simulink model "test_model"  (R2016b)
settings: Solver=VariableStepAuto  StartTime=0.0  StopTime=runtime  RelTol=1e-3
InitFcn:
  | clear mex
  | delete test_model_sfun.mexw64
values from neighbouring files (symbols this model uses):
  g = 9.81    [modelParameters.m]
  height_controlled_o = (((Rm*If +      + (((omega0_o * 2 * Rm * Kv * Kq      * Kd + 1)^2) - 1)/(4* Rm*Kv^2*Kq      * Kd))/Vb)*(Pmax- Pmin) + Pmin)    [modelParameters.m]
  If = 0.511    [modelParameters.m]
  Jreq = 4.2012e-05    [modelParameters.m]
  Jxx = 0.0130    (= 0.013)    [modelParameters.m]
  Jyy = 0.0140    (= 0.014)    [modelParameters.m]
  Jzz = 0.0285    [modelParameters.m]
  Kd = 1.0317e-7    (= 1.0317e-07)    [modelParameters.m]
  Kq = 96.3422    [modelParameters.m]
  Kt = 8.6519e-6    (= 8.6519e-06)    [modelParameters.m]
  Kv = 96.3422    [modelParameters.m]
  m = 1.244    [modelParameters.m]
  omega0_o = sqrt((m*g)/(4*Kt))    [modelParameters.m]
  omega1_o = sqrt((m*g)/(4*Kt))    [modelParameters.m]
  omega2_o = sqrt((m*g)/(4*Kt))    [modelParameters.m]
  omega3_o = sqrt((m*g)/(4*Kt))    [modelParameters.m]
  pitch_o = 0    [modelParameters.m]
  pitchrate_o = 0    [modelParameters.m]
  Pmax = 2e5    (= 200000)    [modelParameters.m]
  Pmin = 1e5    (= 100000)    [modelParameters.m]
  rhx = 0.16    [modelParameters.m]
  rhy = 0.16    [modelParameters.m]
  rhz = 0.03    [modelParameters.m]
  Rm = 0.2308    [modelParameters.m]
  roll_o = 0    [modelParameters.m]
  rollrate_o = 0    [modelParameters.m]
  Tc = 0.04    [modelParameters.m]
  Tq = 0.005    [modelParameters.m]
  Vb = 11.1    [modelParameters.m]
  x_controlled_o = 0    [modelParameters.m]
  x_o = 0    [modelParameters.m]
  x_vel_o = 0    [modelParameters.m]
  y_controlled_o = 0    [modelParameters.m]
  y_o = 0    [modelParameters.m]
  y_vel_o = 0    [modelParameters.m]
  yaw_controlled_o = 0    [modelParameters.m]
  yaw_o = 0    [modelParameters.m]
  yawrate_o = 0    [modelParameters.m]
  z_o = 0    [modelParameters.m]
  z_vel_o = 0    [modelParameters.m]
undefined symbols (not defined in the file or in its folder): DiscIntNeverNeededParam
libraries: simulink x12, vrlib x2
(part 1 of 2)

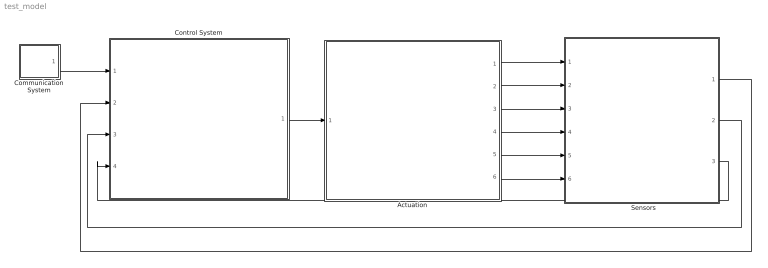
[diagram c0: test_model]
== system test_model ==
  "     Sensors   " : Subsystem
  Actuation : Subsystem
  Communication System : Subsystem
  Control System : Subsystem
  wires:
  Control System/1(P) -> Actuation/1(P)
  Communication System/1(setpoints) -> Control System/1(setpoints)
  Actuation/1(B_omega) -> "     Sensors   "/1(B_Omega)
  Actuation/2(euler_angles) -> "     Sensors   "/2(euler_angles)
  Actuation/3(B_vo) -> "     Sensors   "/3(B_vo)
  Actuation/4(E_ro) -> "     Sensors   "/4(E_ro)
  Actuation/5(B_vo_dot) -> "     Sensors   "/5(B_vo_dot)
  Actuation/6(B_g) -> "     Sensors   "/6(B_g)
  "     Sensors   "/3(current_position) -> Control System/4(current_position)
  "     Sensors   "/2(euler_rates) -> Control System/3(euler_rates)
  "     Sensors   "/1(euler_angles_filtered) -> Control System/2(euler_angles_filtered)

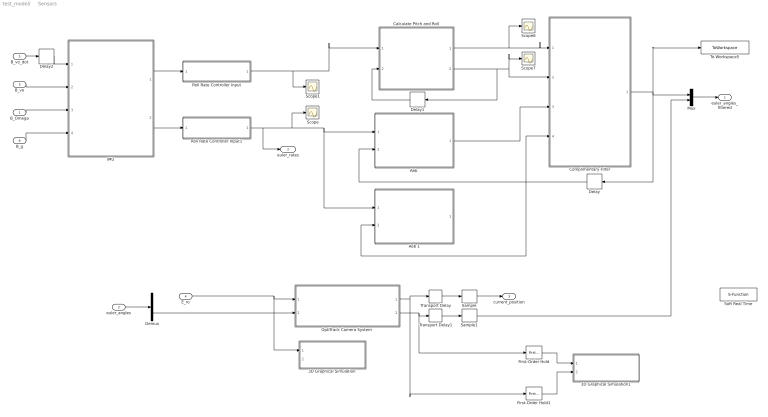
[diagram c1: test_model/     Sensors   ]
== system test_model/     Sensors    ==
  B_Omega : Inport
  euler_angles : Inport  Port=2
  B_vo : Inport  Port=3
  E_ro : Inport  Port=4
  B_vo_dot : Inport  Port=5
  B_g : Inport  Port=6
  3D Graphical Simulation : Subsystem  Commented=on
  3D Graphical Simulation1 : Subsystem  Commented=on
  "Aeb " : MATLAB Function  TreatAsAtomicUnit=on
  Aeb 1 : MATLAB Function  Commented=on  TreatAsAtomicUnit=on
  Calculate Pitch and Roll : MATLAB Function  TreatAsAtomicUnit=on
  Complimentary Filter : MATLAB Function  TreatAsAtomicUnit=on
  Delay : Delay  DelayLength=1  InitialCondition=0
  Delay1 : Delay  DelayLength=1  InitialCondition=0  SampleTime=Tq
  Delay2 : Delay  DelayLength=1  InitialCondition=0  SampleTime=Tq
  Demux : Demux  Outputs=3
  First-Order Hold : simulink/Discrete/First-Order Hold  DisableCoverage=on  Ts=5e-3
  First-Order Hold1 : simulink/Discrete/First-Order Hold  DisableCoverage=on  Ts=5e-3
  "IMU " : Subsystem
  Mux : Mux  Inputs=2
  "OptiTrack Camera System " : Subsystem
  Roll Rate Controller Input : Subsystem  Variant=on
  Roll Rate Controller Input1 : Subsystem  Variant=on
  Sample : ZeroOrderHold  SampleTime=Tc
  Sample1 : ZeroOrderHold  SampleTime=Tc
  Scope{,1,6..7} (4 alike) : Scope
  Soft Real Time : S-Function  Commented=on  FunctionName=sfun_time  Parameters=x  SFunctionDeploymentMode=off  EnableBusSupport=off
  To Workspace5 : ToWorkspace  VariableName=angle_IMU_reading  SaveFormat=Structure With Time  SampleTime=Tq
  Transport Delay : TransportDelay  DelayTime=6e-3
  Transport Delay1 : TransportDelay  DelayTime=6e-3
  euler_angles_filtered : Outport
  euler_rates : Outport  Port=2
  current_position : Outport  Port=3
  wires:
  "IMU "/1(accelerometer) -> Roll Rate Controller Input/1(raw_accel_model)
  "IMU "/2(gyroscope) -> Roll Rate Controller Input1/1(raw_gyro_model)
  B_vo/1 -> "IMU "/2(B_vo)
  B_Omega/1 -> "IMU "/3(B_Omega)
  B_g/1 -> "IMU "/4(B_g)
  Calculate Pitch and Roll/2(accel_roll) -> Scope7/1, Complimentary Filter/2(accel_roll), Delay1/1
  Calculate Pitch and Roll/1(accel_pitch) -> Scope6/1, Complimentary Filter/1(accel_pitch)
  Delay1/1 -> Calculate Pitch and Roll/2(accel_roll_prev)
  First-Order Hold/1 -> 3D Graphical Simulation1/1("Euler Angles ")
  E_ro/1 -> 3D Graphical Simulation/1(Displacement), "OptiTrack Camera System "/1(E_ro)
  First-Order Hold1/1 -> 3D Graphical Simulation1/2(Displacement)
  B_vo_dot/1 -> Delay2/1
  Delay2/1 -> "IMU "/1(B_vo_dot)
  "OptiTrack Camera System "/1(E_ro_camera) -> Transport Delay/1, First-Order Hold1/1
  "OptiTrack Camera System "/2(yaw_camera) -> First-Order Hold/1, Transport Delay1/1
  Transport Delay/1 -> Sample/1
  Transport Delay1/1 -> Sample1/1
  Sample/1 -> current_position/1
  Roll Rate Controller Input/1(raw_accel) -> Calculate Pitch and Roll/1(accel_reading), Scope1/1
  Roll Rate Controller Input1/1(raw_gyro) -> "Aeb "/1(gyro_reading), Aeb 1/1(gyro_reading), Scope/1, euler_rates/1
  Complimentary Filter/1(euler_angles_IMU) -> Mux/1, Delay/1, To Workspace5/1
  Delay/1 -> Aeb 1/2(euler_angles_filtered), Complimentary Filter/4(prev_euler_angles), "Aeb "/2(euler_angles_filtered)
  "Aeb "/1(euler_rates_IMU) -> Complimentary Filter/3(euler_rates_gyro)
  euler_angles/1 -> Demux/1
  Demux/3 -> "OptiTrack Camera System "/2(yaw)
  Sample1/1 -> Mux/2
  Mux/1 -> euler_angles_filtered/1

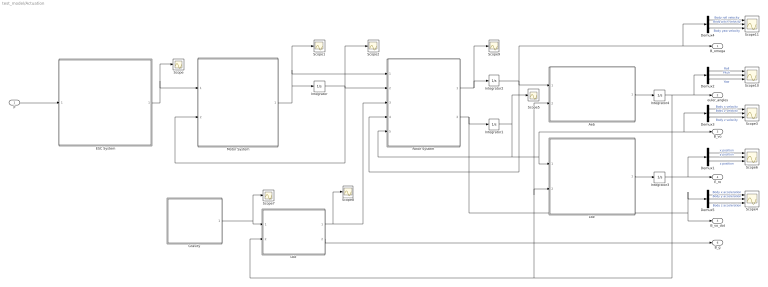
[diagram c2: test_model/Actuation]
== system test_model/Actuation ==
  P : Inport
  "Aeb " : MATLAB Function  TreatAsAtomicUnit=on
  Demux{1..5} (5 alike) : Demux  Outputs=3
  ESC System : MATLAB Function  TreatAsAtomicUnit=on
  "Gravity " : MATLAB Function  TreatAsAtomicUnit=on
  Integrator : Integrator  InitialCondition=[omega0_o, omega1_o, omega2_o, omega3_o]
  Integrator1 : Integrator  InitialCondition=[x_vel_o; y_vel_o; z_vel_o]
  Integrator2 : Integrator  InitialCondition=[rollrate_o; pitchrate_o; yawrate_o]
  Integrator3 : Integrator  InitialCondition=[x_o; y_o; z_o]
  Integrator4 : Integrator  InitialCondition=[roll_o; pitch_o; yaw_o]  ContinuousStateAttributes=['phi' 'theta' 'psi']
  "Lbe " : MATLAB Function  TreatAsAtomicUnit=on
  "Lbe " : MATLAB Function  TreatAsAtomicUnit=on
  Motor System : MATLAB Function  TreatAsAtomicUnit=on
  "Rotor System " : MATLAB Function  TreatAsAtomicUnit=on
  Scope{,1..2,5,7..9} (7 alike) : Scope
  Scope{3..4,6,10..11} (5 alike) : Scope  NumInputPorts=3
  B_omega : Outport
  euler_angles : Outport  Port=2
  B_vo : Outport  Port=3
  E_ro : Outport  Port=4
  B_vo_dot : Outport  Port=5
  B_g : Outport  Port=6
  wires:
  ESC System/1(Vb_eff) -> Scope/1, Motor System/1(Vb_eff)
  Motor System/1(w_dot) -> Integrator/1, "Rotor System "/1(w_dot), Scope1/1
  "Rotor System "/1(B_omega_dot) -> Scope9/1, Integrator2/1
  Integrator2/1 -> "Rotor System "/4(B_omega), B_omega/1, Demux4/1, "Aeb "/1(B_omega)
  "Aeb "/1(euler_rates) -> Integrator4/1
  "Lbe "/1(E_ro) -> Integrator3/1
  Integrator3/1 -> Demux1/1, E_ro/1
  "Lbe "/1(B_Fg) -> Scope8/1, "Rotor System "/3(B_Fg)
  "Lbe "/2(B_g) -> B_g/1
  Demux1/2 -> Scope6/2  "y position"
  Demux1/1 -> Scope6/1  "x position"
  Demux1/3 -> Scope6/3  "z position"
  Demux2/2 -> Scope10/2  "Pitch"
  Demux2/1 -> Scope10/1  "Roll"
  Demux2/3 -> Scope10/3  "Yaw"
  Demux4/2 -> Scope11/2  "Body pitch velocity"
  Demux4/1 -> Scope11/1  "Body roll velocity"
  Demux4/3 -> Scope11/3  "Body yaw velocity"
  Demux3/2 -> Scope3/2  "Body y velocity"
  Demux3/1 -> Scope3/1  "Body x velocity"
  Demux3/3 -> Scope3/3  "Body z velocity"
  Demux5/2 -> Scope4/2  "Body y acceleration"
  Demux5/1 -> Scope4/1  "Body x acceleration"
  Demux5/3 -> Scope4/3  "Body z acceleration"
  Integrator1/1 -> Scope5/1, "Rotor System "/5(B_vo), "Lbe "/1(B_vo), Demux3/1, B_vo/1
  "Rotor System "/2(B_vo_dot) -> Demux5/1, B_vo_dot/1, Integrator1/1
  Integrator4/1 -> euler_angles/1, Demux2/1, "Lbe "/2(euler_angles), "Aeb "/2(euler_angles), "Lbe "/2(euler_angles)
  P/1 -> ESC System/1(P)
  "Gravity "/1(E_Fg) -> Scope7/1, "Lbe "/1(E_Fg)
  Integrator/1 -> Motor System/2(w), "Rotor System "/2(w), Scope2/1

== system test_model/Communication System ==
  Step : Step  Before=[0; 0; 0; 0]  After=[0; 0; 0; 0]  SampleTime=Tq
  setpoints : Outport
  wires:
  Step/1 -> setpoints/1

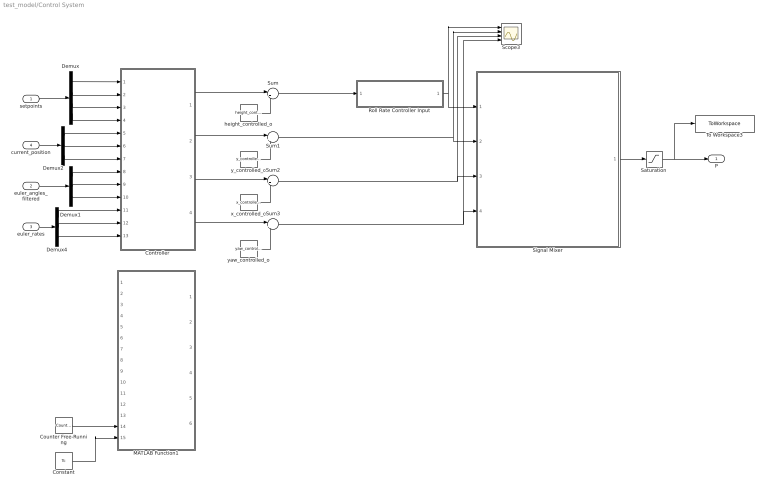
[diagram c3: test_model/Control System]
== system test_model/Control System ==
  setpoints : Inport
  euler_angles_filtered : Inport  Port=2
  euler_rates : Inport  Port=3
  current_position : Inport  Port=4
  Constant : Constant  Value=Tc  SampleTime=Tc
  Controller : Subsystem
  Counter Free-Running : simulink/Sources/Counter Free-Running  NumBits=32  tsamp=Tc
  Demux : Demux
  Demux1 : Demux  Outputs=3
  Demux2 : Demux  Outputs=3
  Demux4 : Demux  Outputs=3
  MATLAB Function1 : MATLAB Function  Commented=on  TreatAsAtomicUnit=on  SystemSampleTime=Tq
  Roll Rate Controller Input : Subsystem  Variant=on
  Saturation : Saturate  UpperLimit=Pmax*ones(4,1)  LowerLimit=Pmin*ones(4,1)
  Scope3 : Scope  NumInputPorts=4
  Signal Mixer : MATLAB Function  TreatAsAtomicUnit=on
  Sum{,1..3} (4 alike) : Sum  Inputs=|++
  To Workspace3 : ToWorkspace  VariableName=motorCommands  SaveFormat=Structure With Time  SampleTime=Tq
  height_controlled_o : Constant  Value=height_controlled_o  SampleTime=Tc
  x_controlled_o : Constant  Value=x_controlled_o
  y_controlled_o : Constant  Value=y_controlled_o
  yaw_controlled_o : Constant  Value=yaw_controlled_o
  P : Outport
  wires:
  setpoints/1 -> Demux/1
  euler_angles_filtered/1 -> Demux1/1
  current_position/1 -> Demux2/1
  euler_rates/1 -> Demux4/1
  Demux/1 -> Controller/1(x_setpoint)
  Demux/2 -> Controller/2(y_setpoint)
  Demux/3 -> Controller/3(z_setpoint)
  Demux2/1 -> Controller/5(x_position)
  Demux2/2 -> Controller/6(y_position)
  Demux2/3 -> Controller/7(z_position)
  Controller/2(y_controlled) -> Sum1/1
  Controller/4(yaw_controlled) -> Sum3/1
  y_controlled_o/1 -> Sum1/2
  x_controlled_o/1 -> Sum2/2
  yaw_controlled_o/1 -> Sum3/2
  Signal Mixer/1(P) -> Saturation/1
  Demux1/1 -> Controller/8(roll)
  Demux1/2 -> Controller/9(pitch)
  Demux4/1 -> Controller/11(roll_rate)
  Demux4/2 -> Controller/12(pitch_rate)
  Demux4/3 -> Controller/13(yaw_rate)
  Demux/4 -> Controller/4(yaw_setpoint)
  Demux1/3 -> Controller/10(yaw)
  Controller/3(x_controlled) -> Sum2/1
  Counter Free-Running/1 -> MATLAB Function1/14(vrpn_id)
  Constant/1 -> MATLAB Function1/15(Tc)
  Sum/1 -> Roll Rate Controller Input/1(z_command_model)
  height_controlled_o/1 -> Sum/2
  Saturation/1 -> To Workspace3/1, P/1
  Sum1/1 -> Scope3/2, Signal Mixer/2(y_controlled)
  Sum2/1 -> Scope3/3, Signal Mixer/3(x_controlled)
  Sum3/1 -> Scope3/4, Signal Mixer/4(yaw_controlled)
  Roll Rate Controller Input/1(z_command) -> Scope3/1, Signal Mixer/1(height_controlled)
  Controller/1(height_controlled) -> Sum/1

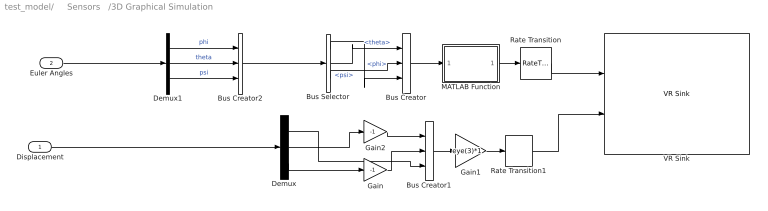
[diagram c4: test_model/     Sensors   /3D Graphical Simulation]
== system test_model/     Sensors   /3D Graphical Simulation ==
  Displacement : Inport
  Euler Angles : Inport  Port=2
  Bus Creator : BusCreator  Inputs=3
  Bus Creator1 : BusCreator  Inputs=3
  Bus Creator2 : BusCreator  Inputs=3
  Bus Selector : BusSelector  OutputSignals=phi,theta,psi
  Demux : Demux  Outputs=3
  Demux1 : Demux  Outputs=3
  Gain : Gain  Gain=-1
  Gain1 : Gain  Gain=eye(3)*1  Multiplication=Matrix(K*u)
  Gain2 : Gain  Gain=-1
  MATLAB Function : MATLAB Function  TreatAsAtomicUnit=on
  Rate Transition : RateTransition  OutPortSampleTime=0.06
  Rate Transition1 : RateTransition  OutPortSampleTime=0.06
  VR Sink : vrlib/VR Sink  InstantiateOnLoad=on  SampleTime=-1  ViewEnable=on  RemoteChange=off  RemoteView=off  FieldsWritten=Helicopter.rotation.4.1.1.double#Helicopter.translation.3.1.1.double  WorldFileName=quadrotor_world_ucart.wrl  AutoView=on  VideoDimensions=[]  AllowVariableSize=off
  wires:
  Displacement/1 -> Demux/1
  Bus Creator2/1 -> Bus Selector/1
  Demux/1 -> Bus Creator1/3
  Gain/1 -> Bus Creator1/2
  Gain2/1 -> Bus Creator1/1
  Rate Transition1/1 -> VR Sink/2
  Rate Transition/1 -> VR Sink/1
  Demux/3 -> Gain/1
  Demux/2 -> Gain2/1
  Bus Creator1/1 -> Gain1/1
  Bus Selector/1 -> Bus Creator/3  "<phi>"
  Bus Selector/3 -> Bus Creator/2  "<psi>"
  Bus Selector/2 -> Bus Creator/1  "<theta>"
  Gain1/1 -> Rate Transition1/1
  Demux1/3 -> Bus Creator2/3  "psi"
  Demux1/2 -> Bus Creator2/2  "theta"
  Demux1/1 -> Bus Creator2/1  "phi"
  Euler Angles/1 -> Demux1/1
  Bus Creator/1 -> MATLAB Function/1(u)
  MATLAB Function/1(y) -> Rate Transition/1

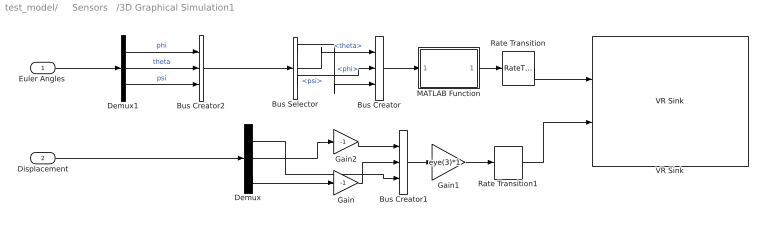
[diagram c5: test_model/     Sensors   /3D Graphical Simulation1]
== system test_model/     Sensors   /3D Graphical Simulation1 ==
  "Euler Angles " : Inport
  Displacement : Inport  Port=2
  Bus Creator : BusCreator  Inputs=3
  Bus Creator1 : BusCreator  Inputs=3
  Bus Creator2 : BusCreator  Inputs=3
  Bus Selector : BusSelector  OutputSignals=phi,theta,psi
  Demux : Demux  Outputs=3
  Demux1 : Demux  Outputs=3
  Gain : Gain  Gain=-1
  Gain1 : Gain  Gain=eye(3)*1  Multiplication=Matrix(K*u)
  Gain2 : Gain  Gain=-1
  MATLAB Function : MATLAB Function  TreatAsAtomicUnit=on
  Rate Transition : RateTransition  OutPortSampleTime=0.06
  Rate Transition1 : RateTransition  OutPortSampleTime=0.06
  VR Sink : vrlib/VR Sink  InstantiateOnLoad=on  SampleTime=-1  ViewEnable=on  RemoteChange=off  RemoteView=off  FieldsWritten=Helicopter.rotation.4.1.1.double#Helicopter.translation.3.1.1.double  WorldFileName=quadrotor_world_ucart.wrl  AutoView=on  VideoDimensions=[]  AllowVariableSize=off
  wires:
  Bus Creator2/1 -> Bus Selector/1
  Demux/1 -> Bus Creator1/3
  Gain/1 -> Bus Creator1/2
  Gain2/1 -> Bus Creator1/1
  Rate Transition1/1 -> VR Sink/2
  Rate Transition/1 -> VR Sink/1
  Demux/3 -> Gain/1
  Demux/2 -> Gain2/1
  Bus Creator1/1 -> Gain1/1
  Bus Selector/1 -> Bus Creator/3  "<phi>"
  Bus Selector/3 -> Bus Creator/2  "<psi>"
  Bus Selector/2 -> Bus Creator/1  "<theta>"
  Gain1/1 -> Rate Transition1/1
  Demux1/3 -> Bus Creator2/3  "psi"
  Demux1/2 -> Bus Creator2/2  "theta"
  Demux1/1 -> Bus Creator2/1  "phi"
  Bus Creator/1 -> MATLAB Function/1(u)
  MATLAB Function/1(y) -> Rate Transition/1
  Displacement/1 -> Demux/1
  "Euler Angles "/1 -> Demux1/1

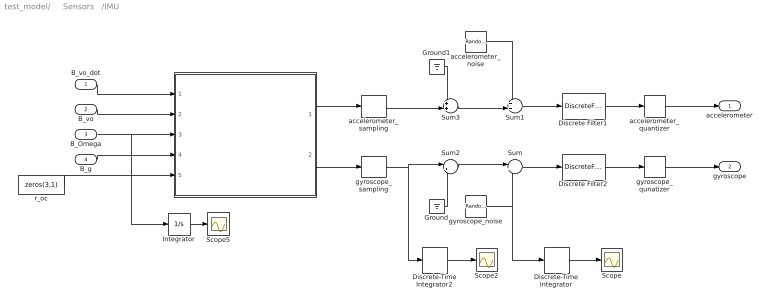
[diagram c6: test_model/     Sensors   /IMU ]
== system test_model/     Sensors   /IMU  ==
  B_vo_dot : Inport
  B_vo : Inport  Port=2
  B_Omega : Inport  Port=3
  B_g : Inport  Port=4
  " " : MATLAB Function  TreatAsAtomicUnit=on
  Discrete Filter1 : DiscreteFilter  Numerator=[0 0.1454]  Denominator=[1 -0.8546]  SampleTime=Tq
  Discrete Filter2 : DiscreteFilter  Numerator=[0 0.1454]  Denominator=[1 -0.8546]  SampleTime=Tq
  Discrete-Time Integrator : DiscreteIntegrator  InitialConditionSetting=State (most efficient)  SampleTime=-1  ICPrevOutput=DiscIntNeverNeededParam  ICPrevScaledInput=DiscIntNeverNeededParam
  Discrete-Time Integrator2 : DiscreteIntegrator  InitialConditionSetting=State (most efficient)  SampleTime=-1  ICPrevOutput=DiscIntNeverNeededParam  ICPrevScaledInput=DiscIntNeverNeededParam
  Ground : Ground
  Ground1 : Ground
  Integrator : Integrator
  Scope : Scope
  Scope2 : Scope
  Scope5 : Scope
  Sum : Sum  Inputs=|++
  Sum1 : Sum  Inputs=++|
  Sum2 : Sum  Inputs=|++
  Sum3 : Sum  Inputs=++|
  accelerometer_noise : RandomNumber  Mean=zeros(3,1)  Variance=[ 3e-7 ; 3.3e-7 ; 7.2e-7 ]  Seed=[0,1,2]  SampleTime=Tq
  accelerometer_quantizer : Quantizer  QuantizationInterval=2.4400e-04
  accelerometer_sampling : ZeroOrderHold  SampleTime=Tq
  gyroscope_noise : RandomNumber  Mean=zeros(3,1)  Variance=[ 2.2e-8 ; 1.1e-7 ; 2.4e-8 ]  Seed=[0,1,2]  SampleTime=Tq
  gyroscope_qunatizer : Quantizer  QuantizationInterval=1.1e-3
  gyroscope_sampling : ZeroOrderHold  SampleTime=Tq
  r_oc : Constant  Value=zeros(3,1)
  accelerometer : Outport
  gyroscope : Outport  Port=2
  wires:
  accelerometer_noise/1 -> Sum1/1
  Sum2/1 -> Sum/1
  Sum3/1 -> Sum1/2
  gyroscope_noise/1 -> Sum/2, Discrete-Time Integrator/1
  gyroscope_sampling/1 -> Sum2/1, Discrete-Time Integrator2/1
  accelerometer_sampling/1 -> Sum3/2
  Ground/1 -> Sum2/2
  Ground1/1 -> Sum3/1
  B_vo_dot/1 -> " "/1(B_vo_dot)
  B_vo/1 -> " "/2(B_vo)
  B_Omega/1 -> Integrator/1, " "/3(B_Omega)
  B_g/1 -> " "/4(B_g)
  r_oc/1 -> " "/5(r_oc)
  " "/2(gyroReading) -> gyroscope_sampling/1
  " "/1(accelReading) -> accelerometer_sampling/1
  Discrete-Time Integrator/1 -> Scope/1
  Discrete-Time Integrator2/1 -> Scope2/1
  Integrator/1 -> Scope5/1
  Sum1/1 -> Discrete Filter1/1
  Sum/1 -> Discrete Filter2/1
  accelerometer_quantizer/1 -> accelerometer/1
  gyroscope_qunatizer/1 -> gyroscope/1
  Discrete Filter1/1 -> accelerometer_quantizer/1
  Discrete Filter2/1 -> gyroscope_qunatizer/1

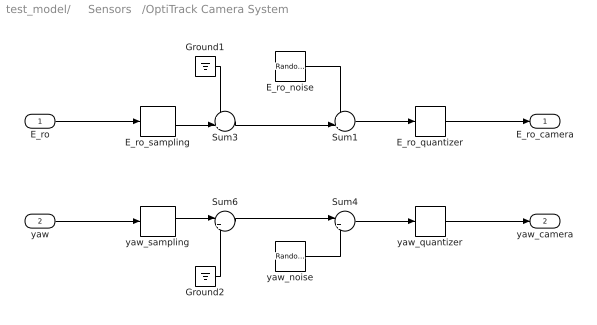
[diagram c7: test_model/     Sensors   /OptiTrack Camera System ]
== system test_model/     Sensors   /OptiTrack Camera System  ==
  E_ro : Inport
  yaw : Inport  Port=2
  E_ro_noise : RandomNumber  Mean=zeros(3,1)  Variance=[ 7.9664e-10 ; 1.1928e-10 ; 5.0636e-10 ]  Seed=[0,1,2]  SampleTime=Tc
  E_ro_quantizer : Quantizer  QuantizationInterval=2.4400e-04
  E_ro_sampling : ZeroOrderHold  SampleTime=Tc
  Ground1 : Ground
  Ground2 : Ground
  Sum1 : Sum  Inputs=++|
  Sum3 : Sum  Inputs=++|
  Sum4 : Sum  Inputs=|++
  Sum6 : Sum  Inputs=|++
  yaw_noise : RandomNumber  Variance=1.0783e-9  SampleTime=Tc
  yaw_quantizer : Quantizer  QuantizationInterval=1.1e-3
  yaw_sampling : ZeroOrderHold  SampleTime=Tc
  E_ro_camera : Outport
  yaw_camera : Outport  Port=2
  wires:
  E_ro_noise/1 -> Sum1/1
  Sum3/1 -> Sum1/2
  Sum1/1 -> E_ro_quantizer/1
  E_ro_sampling/1 -> Sum3/2
  Ground1/1 -> Sum3/1
  Sum4/1 -> yaw_quantizer/1
  Sum6/1 -> Sum4/1
  yaw_noise/1 -> Sum4/2
  yaw_sampling/1 -> Sum6/1
  Ground2/1 -> Sum6/2
  yaw/1 -> yaw_sampling/1
  E_ro/1 -> E_ro_sampling/1
  E_ro_quantizer/1 -> E_ro_camera/1
  yaw_quantizer/1 -> yaw_camera/1

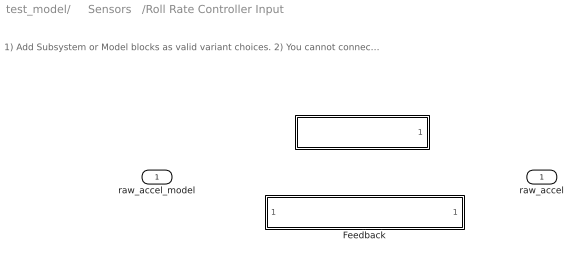
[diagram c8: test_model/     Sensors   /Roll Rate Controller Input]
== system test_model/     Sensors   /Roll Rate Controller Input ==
  note: 1) Add Subsystem or Model blocks as valid variant choices. 2) You cannot connect blocks at this level. At simulation, connectivity is automatically determined, based on the active variant and port name matching.
  raw_accel_model : Inport
  " " : Subsystem  VariantControl=logAnalysisToggle==1
  Feedback : Subsystem  VariantControl=logAnalysisToggle==0
  raw_accel : Outport

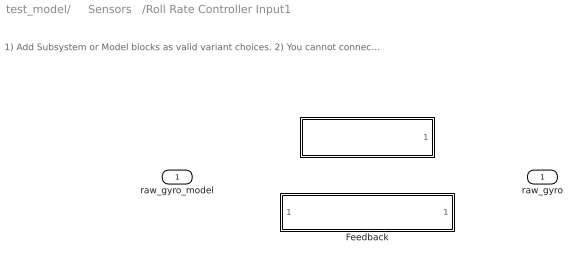
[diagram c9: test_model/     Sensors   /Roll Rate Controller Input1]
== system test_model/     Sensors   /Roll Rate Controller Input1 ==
  note: 1) Add Subsystem or Model blocks as valid variant choices. 2) You cannot connect blocks at this level. At simulation, connectivity is automatically determined, based on the active variant and port name matching.
  raw_gyro_model : Inport
  " " : Subsystem  VariantControl=logAnalysisToggle==1
  Feedback : Subsystem  VariantControl=logAnalysisToggle==0
  raw_gyro : Outport

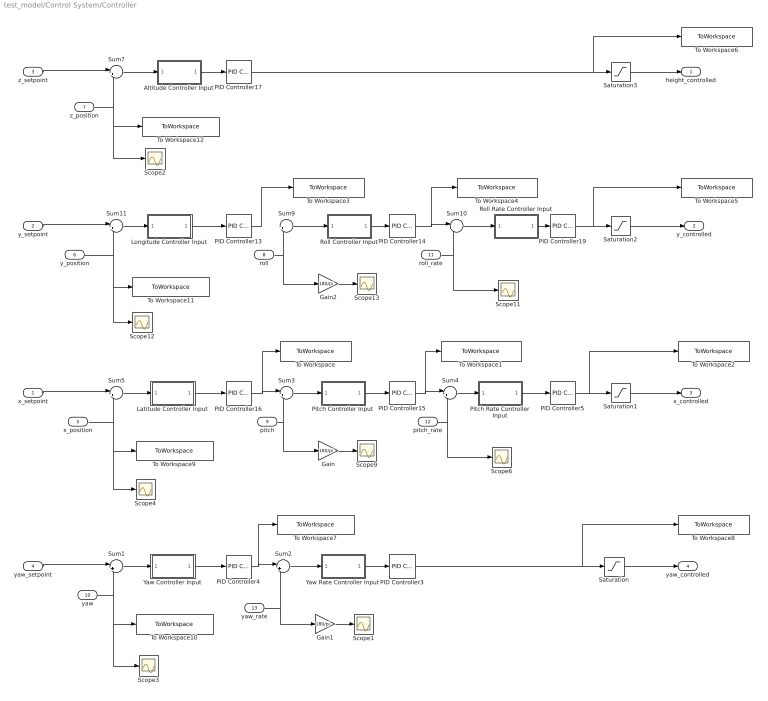
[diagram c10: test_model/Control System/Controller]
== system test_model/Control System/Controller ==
  x_setpoint : Inport
  y_setpoint : Inport  Port=2
  z_setpoint : Inport  Port=3
  yaw_setpoint : Inport  Port=4
  x_position : Inport  Port=5
  y_position : Inport  Port=6
  z_position : Inport  Port=7
  roll : Inport  Port=8
  pitch : Inport  Port=9
  yaw : Inport  Port=10
  roll_rate : Inport  Port=11
  pitch_rate : Inport  Port=12
  yaw_rate : Inport  Port=13
  Altitude Controller Input : Subsystem  Variant=on
  Gain : Gain  Gain=180/pi
  Gain1 : Gain  Gain=180/pi
  Gain2 : Gain  Gain=180/pi
  Latitude Controller Input : Subsystem  Variant=on
  Longitude Controller Input : Subsystem  Variant=on
  PID Controller13 : simulink/Continuous/PID Controller  Controller=PID  TimeDomain=Discrete-time  SampleTime=Tc  IntegratorMethod=Forward Euler  FilterMethod=Forward Euler  Form=Parallel  UseFilter=off  ControllerParametersSource=internal  P=0.015  I=0.005  D=0.03  N=33.9318377685715  InitialConditionSource=internal  InitialConditionForIntegrator=0  InitialConditionForFilter=0  ExternalReset=none  LimitOutput=off  UpperSaturationLimit=inf  LowerSaturationLimit=-inf  LinearizeAsGain=on  AntiWindupMode=none  Kb=1  TrackingMode=off  Kt=1  PParamMin=[]  PParamMax=[]  IParamMin=[]  IParamMax=[]  DParamMin=[]  DParamMax=[]  NParamMin=[]  NParamMax=[]  KbParamMin=[]  KbParamMax=[]  KtParamMin=[]  KtParamMax=[]  POutMin=[]  POutMax=[]  IOutMin=[]  IOutMax=[]  DOutMin=[]  DOutMax=[]  NOutMin=[]  NOutMax=[]  KbOutMin=[]  KbOutMax=[]  KtOutMin=[]  KtOutMax=[]  IntegratorOutMin=[]  IntegratorOutMax=[]  FilterOutMin=[]  FilterOutMax=[]  SumOutMin=[]  SumOutMax=[]  SumI1OutMin=[]  SumI1OutMax=[]  SumI2OutMin=[]  SumI2OutMax=[]  SumI3OutMin=[]  SumI3OutMax=[]  SumDOutMin=[]  SumDOutMax=[]  SaturationOutMin=[]  SaturationOutMax=[]  IntegratorContinuousStateAttributes=''  IntegratorStateMustResolveToSignalObject=off  IntegratorRTWStateStorageClass=Auto  FilterContinuousStateAttributes=''  FilterStateMustResolveToSignalObject=off  FilterRTWStateStorageClass=Auto  DifferentiatorICPrevScaledInput=0  DifferentiatorOutMin=[]  DifferentiatorOutMax=[]
  PID Controller14 : simulink/Continuous/PID Controller  Controller=PD  TimeDomain=Discrete-time  SampleTime=Tq  IntegratorMethod=Forward Euler  FilterMethod=Forward Euler  Form=Parallel  UseFilter=off  ControllerParametersSource=internal  P=15  I=35.1207902652377  D=0.2  N=40.0107970227961  InitialConditionSource=internal  InitialConditionForIntegrator=0  InitialConditionForFilter=0  ExternalReset=none  LimitOutput=off  UpperSaturationLimit=inf  LowerSaturationLimit=-inf  LinearizeAsGain=on  AntiWindupMode=none  Kb=1  TrackingMode=off  Kt=1  PParamMin=[]  PParamMax=[]  IParamMin=[]  IParamMax=[]  DParamMin=[]  DParamMax=[]  NParamMin=[]  NParamMax=[]  KbParamMin=[]  KbParamMax=[]  KtParamMin=[]  KtParamMax=[]  POutMin=[]  POutMax=[]  IOutMin=[]  IOutMax=[]  DOutMin=[]  DOutMax=[]  NOutMin=[]  NOutMax=[]  KbOutMin=[]  KbOutMax=[]  KtOutMin=[]  KtOutMax=[]  IntegratorOutMin=[]  IntegratorOutMax=[]  FilterOutMin=[]  FilterOutMax=[]  SumOutMin=[]  SumOutMax=[]  SumI1OutMin=[]  SumI1OutMax=[]  SumI2OutMin=[]  SumI2OutMax=[]  SumI3OutMin=[]  SumI3OutMax=[]  SumDOutMin=[]  SumDOutMax=[]  SaturationOutMin=[]  SaturationOutMax=[]  IntegratorContinuousStateAttributes=''  IntegratorStateMustResolveToSignalObject=off  IntegratorRTWStateStorageClass=Auto  FilterContinuousStateAttributes=''  FilterStateMustResolveToSignalObject=off  FilterRTWStateStorageClass=Auto  DifferentiatorICPrevScaledInput=0  DifferentiatorOutMin=[]  DifferentiatorOutMax=[]
  PID Controller15 : simulink/Continuous/PID Controller  Controller=PD  TimeDomain=Discrete-time  SampleTime=Tq  IntegratorMethod=Forward Euler  FilterMethod=Forward Euler  Form=Parallel  UseFilter=off  ControllerParametersSource=internal  P=15  I=35.1207902652377  D=0.2  N=40.0107970227961  InitialConditionSource=internal  InitialConditionForIntegrator=0  InitialConditionForFilter=0  ExternalReset=none  LimitOutput=off  UpperSaturationLimit=inf  LowerSaturationLimit=-inf  LinearizeAsGain=on  AntiWindupMode=none  Kb=1  TrackingMode=off  Kt=1  PParamMin=[]  PParamMax=[]  IParamMin=[]  IParamMax=[]  DParamMin=[]  DParamMax=[]  NParamMin=[]  NParamMax=[]  KbParamMin=[]  KbParamMax=[]  KtParamMin=[]  KtParamMax=[]  POutMin=[]  POutMax=[]  IOutMin=[]  IOutMax=[]  DOutMin=[]  DOutMax=[]  NOutMin=[]  NOutMax=[]  KbOutMin=[]  KbOutMax=[]  KtOutMin=[]  KtOutMax=[]  IntegratorOutMin=[]  IntegratorOutMax=[]  FilterOutMin=[]  FilterOutMax=[]  SumOutMin=[]  SumOutMax=[]  SumI1OutMin=[]  SumI1OutMax=[]  SumI2OutMin=[]  SumI2OutMax=[]  SumI3OutMin=[]  SumI3OutMax=[]  SumDOutMin=[]  SumDOutMax=[]  SaturationOutMin=[]  SaturationOutMax=[]  IntegratorContinuousStateAttributes=''  IntegratorStateMustResolveToSignalObject=off  IntegratorRTWStateStorageClass=Auto  FilterContinuousStateAttributes=''  FilterStateMustResolveToSignalObject=off  FilterRTWStateStorageClass=Auto  DifferentiatorICPrevScaledInput=0  DifferentiatorOutMin=[]  DifferentiatorOutMax=[]
  PID Controller16 : simulink/Continuous/PID Controller  Controller=PID  TimeDomain=Discrete-time  SampleTime=Tc  IntegratorMethod=Forward Euler  FilterMethod=Forward Euler  Form=Parallel  UseFilter=off  ControllerParametersSource=internal  P=-0.015  I=-0.005  D=-0.03  N=33.9318377685715  InitialConditionSource=internal  InitialConditionForIntegrator=0  InitialConditionForFilter=0  ExternalReset=none  LimitOutput=off  UpperSaturationLimit=inf  LowerSaturationLimit=-inf  LinearizeAsGain=on  AntiWindupMode=none  Kb=1  TrackingMode=off  Kt=1  PParamMin=[]  PParamMax=[]  IParamMin=[]  IParamMax=[]  DParamMin=[]  DParamMax=[]  NParamMin=[]  NParamMax=[]  KbParamMin=[]  KbParamMax=[]  KtParamMin=[]  KtParamMax=[]  POutMin=[]  POutMax=[]  IOutMin=[]  IOutMax=[]  DOutMin=[]  DOutMax=[]  NOutMin=[]  NOutMax=[]  KbOutMin=[]  KbOutMax=[]  KtOutMin=[]  KtOutMax=[]  IntegratorOutMin=[]  IntegratorOutMax=[]  FilterOutMin=[]  FilterOutMax=[]  SumOutMin=[]  SumOutMax=[]  SumI1OutMin=[]  SumI1OutMax=[]  SumI2OutMin=[]  SumI2OutMax=[]  SumI3OutMin=[]  SumI3OutMax=[]  SumDOutMin=[]  SumDOutMax=[]  SaturationOutMin=[]  SaturationOutMax=[]  IntegratorContinuousStateAttributes=''  IntegratorStateMustResolveToSignalObject=off  IntegratorRTWStateStorageClass=Auto  FilterContinuousStateAttributes=''  FilterStateMustResolveToSignalObject=off  FilterRTWStateStorageClass=Auto  DifferentiatorICPrevScaledInput=0  DifferentiatorOutMin=[]  DifferentiatorOutMax=[]
  PID Controller17 : simulink/Continuous/PID Controller  Controller=PID  TimeDomain=Discrete-time  SampleTime=Tc  IntegratorMethod=Forward Euler  FilterMethod=Forward Euler  Form=Parallel  UseFilter=off  ControllerParametersSource=internal  P=9804  I=817  D=7353  N=5.79502261645411  InitialConditionSource=internal  InitialConditionForIntegrator=0  InitialConditionForFilter=0  ExternalReset=none  LimitOutput=off  UpperSaturationLimit=inf  LowerSaturationLimit=-inf  LinearizeAsGain=on  AntiWindupMode=none  Kb=1  TrackingMode=off  Kt=1  PParamMin=[]  PParamMax=[]  IParamMin=[]  IParamMax=[]  DParamMin=[]  DParamMax=[]  NParamMin=[]  NParamMax=[]  KbParamMin=[]  KbParamMax=[]  KtParamMin=[]  KtParamMax=[]  POutMin=[]  POutMax=[]  IOutMin=[]  IOutMax=[]  DOutMin=[]  DOutMax=[]  NOutMin=[]  NOutMax=[]  KbOutMin=[]  KbOutMax=[]  KtOutMin=[]  KtOutMax=[]  IntegratorOutMin=[]  IntegratorOutMax=[]  FilterOutMin=[]  FilterOutMax=[]  SumOutMin=[]  SumOutMax=[]  SumI1OutMin=[]  SumI1OutMax=[]  SumI2OutMin=[]  SumI2OutMax=[]  SumI3OutMin=[]  SumI3OutMax=[]  SumDOutMin=[]  SumDOutMax=[]  SaturationOutMin=[]  SaturationOutMax=[]  IntegratorContinuousStateAttributes=''  IntegratorStateMustResolveToSignalObject=off  IntegratorRTWStateStorageClass=Auto  FilterContinuousStateAttributes=''  FilterStateMustResolveToSignalObject=off  FilterRTWStateStorageClass=Auto  DifferentiatorICPrevScaledInput=0  DifferentiatorOutMin=[]  DifferentiatorOutMax=[]
  PID Controller19 : simulink/Continuous/PID Controller  Controller=PD  TimeDomain=Discrete-time  SampleTime=Tq  IntegratorMethod=Forward Euler  FilterMethod=Forward Euler  Form=Parallel  UseFilter=off  ControllerParametersSource=internal  P=4600  I=1575.82088970639  D=550  N=244.660686071579  InitialConditionSource=internal  InitialConditionForIntegrator=0  InitialConditionForFilter=0  ExternalReset=none  LimitOutput=off  UpperSaturationLimit=inf  LowerSaturationLimit=-inf  LinearizeAsGain=on  AntiWindupMode=none  Kb=1  TrackingMode=off  Kt=1  PParamMin=[]  PParamMax=[]  IParamMin=[]  IParamMax=[]  DParamMin=[]  DParamMax=[]  NParamMin=[]  NParamMax=[]  KbParamMin=[]  KbParamMax=[]  KtParamMin=[]  KtParamMax=[]  POutMin=[]  POutMax=[]  IOutMin=[]  IOutMax=[]  DOutMin=[]  DOutMax=[]  NOutMin=[]  NOutMax=[]  KbOutMin=[]  KbOutMax=[]  KtOutMin=[]  KtOutMax=[]  IntegratorOutMin=[]  IntegratorOutMax=[]  FilterOutMin=[]  FilterOutMax=[]  SumOutMin=[]  SumOutMax=[]  SumI1OutMin=[]  SumI1OutMax=[]  SumI2OutMin=[]  SumI2OutMax=[]  SumI3OutMin=[]  SumI3OutMax=[]  SumDOutMin=[]  SumDOutMax=[]  SaturationOutMin=[]  SaturationOutMax=[]  IntegratorContinuousStateAttributes=''  IntegratorStateMustResolveToSignalObject=off  IntegratorRTWStateStorageClass=Auto  FilterContinuousStateAttributes=''  FilterStateMustResolveToSignalObject=off  FilterRTWStateStorageClass=Auto  DifferentiatorICPrevScaledInput=0  DifferentiatorOutMin=[]  DifferentiatorOutMax=[]
  PID Controller3 : simulink/Continuous/PID Controller  Controller=P  TimeDomain=Discrete-time  SampleTime=Tq  IntegratorMethod=Forward Euler  FilterMethod=Forward Euler  Form=Parallel  UseFilter=on  ControllerParametersSource=internal  P=435480  I=-77.7  D=2.32  N=1/0.0818  InitialConditionSource=internal  InitialConditionForIntegrator=0  InitialConditionForFilter=0  ExternalReset=none  ZeroCross=off  LimitOutput=off  UpperSaturationLimit=inf  LowerSaturationLimit=-inf  LinearizeAsGain=on  AntiWindupMode=none  Kb=1  TrackingMode=off  Kt=1  PParamMin=[]  PParamMax=[]  IParamMin=[]  IParamMax=[]  DParamMin=[]  DParamMax=[]  NParamMin=[]  NParamMax=[]  KbParamMin=[]  KbParamMax=[]  KtParamMin=[]  KtParamMax=[]  POutMin=[]  POutMax=[]  IOutMin=[]  IOutMax=[]  DOutMin=[]  DOutMax=[]  NOutMin=[]  NOutMax=[]  KbOutMin=[]  KbOutMax=[]  KtOutMin=[]  KtOutMax=[]  IntegratorOutMin=[]  IntegratorOutMax=[]  FilterOutMin=[]  FilterOutMax=[]  SumOutMin=[]  SumOutMax=[]  SumI1OutMin=[]  SumI1OutMax=[]  SumI2OutMin=[]  SumI2OutMax=[]  SumI3OutMin=[]  SumI3OutMax=[]  SumDOutMin=[]  SumDOutMax=[]  SaturationOutMin=[]  SaturationOutMax=[]  IntegratorContinuousStateAttributes=''  IntegratorStateMustResolveToSignalObject=off  IntegratorRTWStateStorageClass=Auto  FilterContinuousStateAttributes=''  FilterStateMustResolveToSignalObject=off  FilterRTWStateStorageClass=Auto  DifferentiatorICPrevScaledInput=0  DifferentiatorOutMin=[]  DifferentiatorOutMax=[]
  PID Controller4 : simulink/Continuous/PID Controller  Controller=PD  TimeDomain=Discrete-time  SampleTime=Tc  IntegratorMethod=Forward Euler  FilterMethod=Forward Euler  Form=Parallel  UseFilter=off  ControllerParametersSource=internal  P=2.6  I=2.36803176515497  D=0  N=3.83298618768959  InitialConditionSource=internal  InitialConditionForIntegrator=0  InitialConditionForFilter=0  ExternalReset=none  LimitOutput=off  UpperSaturationLimit=inf  LowerSaturationLimit=-inf  LinearizeAsGain=on  AntiWindupMode=none  Kb=1  TrackingMode=off  Kt=1  PParamMin=[]  PParamMax=[]  IParamMin=[]  IParamMax=[]  DParamMin=[]  DParamMax=[]  NParamMin=[]  NParamMax=[]  KbParamMin=[]  KbParamMax=[]  KtParamMin=[]  KtParamMax=[]  POutMin=[]  POutMax=[]  IOutMin=[]  IOutMax=[]  DOutMin=[]  DOutMax=[]  NOutMin=[]  NOutMax=[]  KbOutMin=[]  KbOutMax=[]  KtOutMin=[]  KtOutMax=[]  IntegratorOutMin=[]  IntegratorOutMax=[]  FilterOutMin=[]  FilterOutMax=[]  SumOutMin=[]  SumOutMax=[]  SumI1OutMin=[]  SumI1OutMax=[]  SumI2OutMin=[]  SumI2OutMax=[]  SumI3OutMin=[]  SumI3OutMax=[]  SumDOutMin=[]  SumDOutMax=[]  SaturationOutMin=[]  SaturationOutMax=[]  IntegratorContinuousStateAttributes=''  IntegratorStateMustResolveToSignalObject=off  IntegratorRTWStateStorageClass=Auto  FilterContinuousStateAttributes=''  FilterStateMustResolveToSignalObject=off  FilterRTWStateStorageClass=Auto  DifferentiatorICPrevScaledInput=0  DifferentiatorOutMin=[]  DifferentiatorOutMax=[]
  PID Controller5 : simulink/Continuous/PID Controller  Controller=PD  TimeDomain=Discrete-time  SampleTime=Tq  IntegratorMethod=Forward Euler  FilterMethod=Forward Euler  Form=Parallel  UseFilter=off  ControllerParametersSource=internal  P=4600  I=1575.82088970639  D=550  N=244.660686071579  InitialConditionSource=internal  InitialConditionForIntegrator=0  InitialConditionForFilter=0  ExternalReset=none  LimitOutput=off  UpperSaturationLimit=inf  LowerSaturationLimit=-inf  LinearizeAsGain=on  AntiWindupMode=none  Kb=1  TrackingMode=off  Kt=1  PParamMin=[]  PParamMax=[]  IParamMin=[]  IParamMax=[]  DParamMin=[]  DParamMax=[]  NParamMin=[]  NParamMax=[]  KbParamMin=[]  KbParamMax=[]  KtParamMin=[]  KtParamMax=[]  POutMin=[]  POutMax=[]  IOutMin=[]  IOutMax=[]  DOutMin=[]  DOutMax=[]  NOutMin=[]  NOutMax=[]  KbOutMin=[]  KbOutMax=[]  KtOutMin=[]  KtOutMax=[]  IntegratorOutMin=[]  IntegratorOutMax=[]  FilterOutMin=[]  FilterOutMax=[]  SumOutMin=[]  SumOutMax=[]  SumI1OutMin=[]  SumI1OutMax=[]  SumI2OutMin=[]  SumI2OutMax=[]  SumI3OutMin=[]  SumI3OutMax=[]  SumDOutMin=[]  SumDOutMax=[]  SaturationOutMin=[]  SaturationOutMax=[]  IntegratorContinuousStateAttributes=''  IntegratorStateMustResolveToSignalObject=off  IntegratorRTWStateStorageClass=Auto  FilterContinuousStateAttributes=''  FilterStateMustResolveToSignalObject=off  FilterRTWStateStorageClass=Auto  DifferentiatorICPrevScaledInput=0  DifferentiatorOutMin=[]  DifferentiatorOutMax=[]
  Pitch Controller Input : Subsystem  Variant=on
  Pitch Rate Controller Input : Subsystem  Variant=on
  Roll Controller Input : Subsystem  Variant=on
  Roll Rate Controller Input : Subsystem  Variant=on
  Saturation{,1..3} (4 alike) : Saturate  UpperLimit=30000  LowerLimit=-30000
  Scope{1..4,6,9,11..13} (9 alike) : Scope
  Sum{1..5,7,9..11} (9 alike) : Sum  Inputs=|+-
  To Workspace : ToWorkspace  VariableName=pitch_setpoint_model  SaveFormat=Structure With Time  SampleTime=-1
  To Workspace1 : ToWorkspace  VariableName=pitchrate_setpoint_model  SaveFormat=Structure With Time  SampleTime=Tq
  To Workspace10 : ToWorkspace  VariableName=yaw_value_model  SaveFormat=Structure With Time  SampleTime=Tc
  To Workspace11 : ToWorkspace  VariableName=y_position_model  SaveFormat=Structure With Time  SampleTime=Tc
  To Workspace12 : ToWorkspace  VariableName=z_position_model  SaveFormat=Structure With Time  SampleTime=Tc
  To Workspace2 : ToWorkspace  VariableName=x_command_model  SaveFormat=Structure With Time  SampleTime=Tq
  To Workspace3 : ToWorkspace  VariableName=roll_setpoint_model  SaveFormat=Structure With Time  SampleTime=Tc
  To Workspace4 : ToWorkspace  VariableName=rollrate_setpoint_model  SaveFormat=Structure With Time  SampleTime=Tq
  To Workspace5 : ToWorkspace  VariableName=y_command_model  SaveFormat=Structure With Time  SampleTime=Tq
  To Workspace6 : ToWorkspace  VariableName=z_command_model  SaveFormat=Structure With Time  SampleTime=Tc
  To Workspace7 : ToWorkspace  VariableName=yawrate_setpoint_model  SaveFormat=Structure With Time  SampleTime=Tc
  To Workspace8 : ToWorkspace  VariableName=yaw_command_model  SaveFormat=Structure With Time  SampleTime=Tq
  To Workspace9 : ToWorkspace  VariableName=x_position_model  SaveFormat=Structure With Time  SampleTime=Tc
  Yaw Controller Input : Subsystem  Variant=on
  Yaw Rate Controller Input : Subsystem  Variant=on
  height_controlled : Outport
  y_controlled : Outport  Port=2
  x_controlled : Outport  Port=3
  yaw_controlled : Outport  Port=4
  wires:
  pitch_rate/1 -> Scope6/1, Sum4/2
  z_setpoint/1 -> Sum7/1
  x_position/1 -> Scope4/1, To Workspace9/1, Sum5/2
  PID Controller15/1 -> Sum4/1, To Workspace1/1
  PID Controller16/1 -> Sum3/1, To Workspace/1
  pitch/1 -> Gain/1, Sum3/2
  Gain/1 -> Scope9/1
  PID Controller3/1 -> To Workspace8/1, Saturation/1
  PID Controller5/1 -> To Workspace2/1, Saturation1/1
  Latitude Controller Input/1(x_error) -> PID Controller16/1
  x_setpoint/1 -> Sum5/1
  roll_rate/1 -> Scope11/1, Sum10/2
  y_position/1 -> Scope12/1, To Workspace11/1, Sum11/2
  PID Controller14/1 -> Sum10/1, To Workspace4/1
  PID Controller13/1 -> To Workspace3/1
  roll/1 -> Gain2/1, Sum9/2
  Gain2/1 -> Scope13/1
  PID Controller19/1 -> To Workspace5/1, Saturation2/1
  y_setpoint/1 -> Sum11/1
  PID Controller17/1 -> To Workspace6/1, Saturation3/1
  yaw/1 -> Scope3/1, To Workspace10/1, Sum1/2
  yaw_setpoint/1 -> Sum1/1
  yaw_rate/1 -> Gain1/1, Sum2/2
  Gain1/1 -> Scope1/1
  PID Controller4/1 -> To Workspace7/1, Sum2/1
  z_position/1 -> To Workspace12/1, Scope2/1, Sum7/2
  Sum1/1 -> Yaw Controller Input/1(yaw_error_model)
  Yaw Controller Input/1(yaw_error) -> PID Controller4/1
  Sum2/1 -> Yaw Rate Controller Input/1(yawrate_error_model)
  Yaw Rate Controller Input/1(yawrate_error) -> PID Controller3/1
  Sum5/1 -> Latitude Controller Input/1(x_error_model)
  Sum3/1 -> Pitch Controller Input/1(pitch_error_model)
  Pitch Controller Input/1(pitch_error) -> PID Controller15/1
  Sum4/1 -> Pitch Rate Controller Input/1(pitchrate_error_model)
  Pitch Rate Controller Input/1(pitchrate_error) -> PID Controller5/1
  Sum11/1 -> Longitude Controller Input/1(y_error_model)
  Longitude Controller Input/1(y_error) -> PID Controller13/1
  Sum9/1 -> Roll Controller Input/1(roll_error_model)
  Roll Controller Input/1(roll_error) -> PID Controller14/1
  Sum10/1 -> Roll Rate Controller Input/1(rollrate_error_model)
  Roll Rate Controller Input/1(rollrate_error) -> PID Controller19/1
  Altitude Controller Input/1(z_error) -> PID Controller17/1
  Sum7/1 -> Altitude Controller Input/1(z_error_model)
  Saturation2/1 -> y_controlled/1
  Saturation3/1 -> height_controlled/1
  Saturation1/1 -> x_controlled/1
  Saturation/1 -> yaw_controlled/1

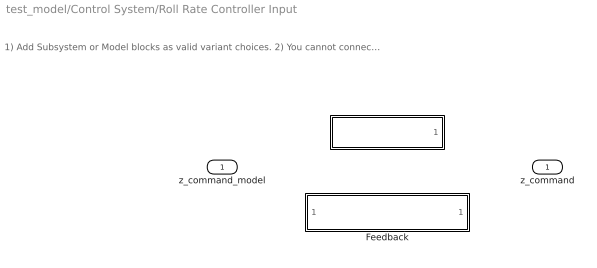
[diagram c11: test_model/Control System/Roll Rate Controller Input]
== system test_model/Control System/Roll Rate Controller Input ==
  note: 1) Add Subsystem or Model blocks as valid variant choices. 2) You cannot connect blocks at this level. At simulation, connectivity is automatically determined, based on the active variant and port name matching.
  z_command_model : Inport
  " " : Subsystem  VariantControl=logAnalysisToggle==1
  Feedback : Subsystem  VariantControl=logAnalysisToggle==0
  z_command : Outport

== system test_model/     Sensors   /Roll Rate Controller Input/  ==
  From Workspace5 : FromWorkspace  VariableName=raw_accel_data  SampleTime=Tq
  raw_accel : Outport
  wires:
  From Workspace5/1 -> raw_accel/1

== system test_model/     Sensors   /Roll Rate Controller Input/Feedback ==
  raw_accel_model : Inport
  raw_accel : Outport
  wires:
  raw_accel_model/1 -> raw_accel/1

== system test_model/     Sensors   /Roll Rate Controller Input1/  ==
  From Workspace5 : FromWorkspace  VariableName=raw_accel_data  SampleTime=Tq
  raw_gyro : Outport
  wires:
  From Workspace5/1 -> raw_gyro/1

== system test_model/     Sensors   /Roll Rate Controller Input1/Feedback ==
  raw_gyro_model : Inport
  raw_gyro : Outport
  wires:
  raw_gyro_model/1 -> raw_gyro/1

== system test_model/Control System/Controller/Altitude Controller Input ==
  note: 1) Add Subsystem or Model blocks as valid variant choices. 2) You cannot connect blocks at this level. At simulation, connectivity is automatically determined, based on the active variant and port name matching.
  z_error_model : Inport
  Feedback : Subsystem  VariantControl=logAnalysisToggle==0
  z error : Subsystem  VariantControl=logAnalysisToggle==1
  z_error : Outport

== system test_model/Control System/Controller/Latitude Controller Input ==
  note: 1) Add Subsystem or Model blocks as valid variant choices. 2) You cannot connect blocks at this level. At simulation, connectivity is automatically determined, based on the active variant and port name matching.
  x_error_model : Inport
  Feedback : Subsystem  VariantControl=logAnalysisToggle==0
  x error : Subsystem  VariantControl=logAnalysisToggle==1
  x_error : Outport

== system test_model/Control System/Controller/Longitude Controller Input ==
  note: 1) Add Subsystem or Model blocks as valid variant choices. 2) You cannot connect blocks at this level. At simulation, connectivity is automatically determined, based on the active variant and port name matching.
  y_error_model : Inport
  Feedback : Subsystem  VariantControl=logAnalysisToggle==0
  y error : Subsystem  VariantControl=logAnalysisToggle==1
  y_error : Outport

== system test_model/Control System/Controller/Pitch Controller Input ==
  note: 1) Add Subsystem or Model blocks as valid variant choices. 2) You cannot connect blocks at this level. At simulation, connectivity is automatically determined, based on the active variant and port name matching.
  pitch_error_model : Inport
  Feedback : Subsystem  VariantControl=logAnalysisToggle==0
  pitch error : Subsystem  VariantControl=logAnalysisToggle==1
  pitch_error : Outport

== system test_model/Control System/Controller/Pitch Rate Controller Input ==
  note: 1) Add Subsystem or Model blocks as valid variant choices. 2) You cannot connect blocks at this level. At simulation, connectivity is automatically determined, based on the active variant and port name matching.
  pitchrate_error_model : Inport
  Feedback : Subsystem  VariantControl=logAnalysisToggle==0
  pitchrate error : Subsystem  VariantControl=logAnalysisToggle==1
  pitchrate_error : Outport

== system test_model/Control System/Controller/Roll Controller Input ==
  note: 1) Add Subsystem or Model blocks as valid variant choices. 2) You cannot connect blocks at this level. At simulation, connectivity is automatically determined, based on the active variant and port name matching.
  roll_error_model : Inport
  Feedback : Subsystem  VariantControl=logAnalysisToggle==0
  roll error : Subsystem  VariantControl=logAnalysisToggle==1
  roll_error : Outport

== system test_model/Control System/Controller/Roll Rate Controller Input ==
  note: 1) Add Subsystem or Model blocks as valid variant choices. 2) You cannot connect blocks at this level. At simulation, connectivity is automatically determined, based on the active variant and port name matching.
  rollrate_error_model : Inport
  Feedback : Subsystem  VariantControl=logAnalysisToggle==0
  rollrate error : Subsystem  VariantControl=logAnalysisToggle==1
  rollrate_error : Outport

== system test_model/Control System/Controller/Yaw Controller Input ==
  note: 1) Add Subsystem or Model blocks as valid variant choices. 2) You cannot connect blocks at this level. At simulation, connectivity is automatically determined, based on the active variant and port name matching.
  yaw_error_model : Inport
  Feedback : Subsystem  VariantControl=logAnalysisToggle==0
  yaw error : Subsystem  VariantControl=logAnalysisToggle==1
  yaw_error : Outport

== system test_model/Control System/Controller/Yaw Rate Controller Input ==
  note: 1) Add Subsystem or Model blocks as valid variant choices. 2) You cannot connect blocks at this level. At simulation, connectivity is automatically determined, based on the active variant and port name matching.
  yawrate_error_model : Inport
  Feedback : Subsystem  VariantControl=logAnalysisToggle==0
  yawrate error : Subsystem  VariantControl=logAnalysisToggle==1
  yawrate_error : Outport

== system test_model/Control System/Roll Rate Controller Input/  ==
  From Workspace5 : FromWorkspace  VariableName=throttle_command  SampleTime=Tq
  z_command : Outport
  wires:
  From Workspace5/1 -> z_command/1

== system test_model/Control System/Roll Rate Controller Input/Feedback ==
  z_command_model : Inport
  z_command : Outport
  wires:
  z_command_model/1 -> z_command/1

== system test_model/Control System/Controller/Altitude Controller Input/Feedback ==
  z_error_model : Inport
  z_error : Outport
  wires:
  z_error_model/1 -> z_error/1

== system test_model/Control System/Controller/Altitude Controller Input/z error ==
  From Workspace6 : FromWorkspace  VariableName=z_error  SampleTime=Tc
  z_error : Outport
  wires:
  From Workspace6/1 -> z_error/1

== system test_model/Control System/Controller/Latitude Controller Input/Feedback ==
  x_error_model : Inport
  x_error : Outport
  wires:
  x_error_model/1 -> x_error/1

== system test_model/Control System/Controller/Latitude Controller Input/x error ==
  From Workspace : FromWorkspace  VariableName=x_error  SampleTime=Tc
  x_error : Outport
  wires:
  From Workspace/1 -> x_error/1

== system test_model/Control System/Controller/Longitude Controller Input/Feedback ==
  y_error_model : Inport
  y_error : Outport
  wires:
  y_error_model/1 -> y_error/1

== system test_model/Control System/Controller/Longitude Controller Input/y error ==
  From Workspace3 : FromWorkspace  VariableName=y_error  SampleTime=Tc
  y_error : Outport
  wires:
  From Workspace3/1 -> y_error/1

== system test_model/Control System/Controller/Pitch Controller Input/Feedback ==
  pitch_error_model : Inport
  pitch_error : Outport
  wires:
  pitch_error_model/1 -> pitch_error/1

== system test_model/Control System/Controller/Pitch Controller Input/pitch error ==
  From Workspace : FromWorkspace  VariableName=pitch_error  SampleTime=Tq
  pitch_error : Outport
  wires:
  From Workspace/1 -> pitch_error/1

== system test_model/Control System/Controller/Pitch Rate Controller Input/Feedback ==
  pitchrate_error_model : Inport
  pitchrate_error : Outport
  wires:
  pitchrate_error_model/1 -> pitchrate_error/1

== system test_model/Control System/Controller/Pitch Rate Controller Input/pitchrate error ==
  From Workspace2 : FromWorkspace  VariableName=pitchrate_error  SampleTime=Tq
  pitchrate_error : Outport
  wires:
  From Workspace2/1 -> pitchrate_error/1

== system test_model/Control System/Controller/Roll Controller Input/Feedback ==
  roll_error_model : Inport
  roll_error : Outport
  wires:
  roll_error_model/1 -> roll_error/1

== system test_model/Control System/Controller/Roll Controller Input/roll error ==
  From Workspace4 : FromWorkspace  VariableName=roll_error  SampleTime=Tq
  roll_error : Outport
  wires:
  From Workspace4/1 -> roll_error/1

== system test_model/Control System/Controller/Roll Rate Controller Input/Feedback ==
  rollrate_error_model : Inport
  rollrate_error : Outport
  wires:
  rollrate_error_model/1 -> rollrate_error/1

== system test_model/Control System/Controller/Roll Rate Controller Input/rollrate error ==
  From Workspace5 : FromWorkspace  VariableName=rollrate_error  SampleTime=Tq
  rollrate_error : Outport
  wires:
  From Workspace5/1 -> rollrate_error/1

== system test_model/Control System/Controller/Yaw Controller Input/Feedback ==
  yaw_error_model : Inport
  yaw_error : Outport
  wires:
  yaw_error_model/1 -> yaw_error/1

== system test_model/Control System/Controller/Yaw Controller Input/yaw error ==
  From Workspace7 : FromWorkspace  VariableName=yaw_error  SampleTime=Tc
  yaw_error : Outport
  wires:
  From Workspace7/1 -> yaw_error/1

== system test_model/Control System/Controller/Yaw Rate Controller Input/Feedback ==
  yawrate_error_model : Inport
  yawrate_error : Outport
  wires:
  yawrate_error_model/1 -> yawrate_error/1

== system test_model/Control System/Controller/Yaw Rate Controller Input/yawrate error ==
  From Workspace8 : FromWorkspace  VariableName=yawrate_error  SampleTime=Tq
  yawrate_error : Outport
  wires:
  From Workspace8/1 -> yawrate_error/1

== matlab function test_model/Actuation/Gravity

 ==
function E_Fg = gravity(m, g)

E_Fg = [0; 0; m*g];

== matlab function test_model/Actuation/Lbe





 ==
function E_ro  = linear_body_earth_conversion(B_vo, euler_angles)

euler_rates = zeros(3,1);
E_ro = zeros(3,1);

phi = euler_angles(1);
theta = euler_angles(2);
psi = euler_angles(3);

Leb = [cos(theta)*cos(psi), sin(phi)*sin(theta)*cos(psi)-cos(phi)*sin(psi), cos(phi)*sin(theta)*cos(psi)+sin(phi)*sin(psi); ...
       cos(theta)*sin(psi), sin(phi)*sin(theta)*sin(psi)+cos(phi)*cos(psi), cos(phi)*sin(theta)*sin(psi)-sin(phi)*cos(psi); ...
           -sin(theta)    ,                sin(phi)*cos(theta)            ,                 cos(phi)*cos(theta)           ];

E_ro = Leb * B_vo;

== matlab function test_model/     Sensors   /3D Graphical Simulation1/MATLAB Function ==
function y = eigenaxis_ucart(u)


if abs(u(1))< 0.0001
    u(1) = 0.0001;
end

if abs(u(2))< 0.0001
    u(2) = 0.0001;
end

if abs(u(3))< 0.0001
    u(3) = 0.0001;
end

u = [ -u(1); -u(2); u(3) ];% [Pitch, Yaw, Roll] 

C11 = cos(u(2))*cos(u(3));
C12 = cos(u(2))*sin(u(3));
C13 = -sin(u(2));
C21 = sin(u(1))*sin(u(2))*cos(u(3))-cos(u(1))*sin(u(3));
C22 = sin(u(1))*sin(u(2))*sin(u(3))+cos(u(1))*cos(u(3));
C23 = sin(u(1))*cos(u(2));
C31 = cos(u(1))*sin(u(2))*cos(u(3))+sin(u(1))*sin(u(3));
C32 = cos(u(1))*sin(u(2))*sin(u(3))-sin(u(1))*cos(u(3));
C33 = cos(u(1))*cos(u(2));
    
theta = acos(0.5*(C11+C22+C33-1));

e = [C23-C32; C31-C13; C12-C21]/(2*sin(theta));
    
y = [e; theta];

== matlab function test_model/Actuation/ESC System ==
function Vb_eff   = ESC(P, Pmin, Pmax, Vb)

P1 = P(1);
P2 = P(2);
P3 = P(3);
P4 = P(4);

% Define u_Pi for each of the rotors, limiting it to be greater than 0
% u_P0 = (rotor_0_duty_cycle/100 - Pmin) / (Pmax - Pmin);
% u_P1 = (rotor_1_duty_cycle/100 - Pmin) / (Pmax - Pmin);
% u_P2 = (rotor_2_duty_cycle/100 - Pmin) / (Pmax - Pmin);
% u_P3 = (rotor_3_duty_cycle/100 - Pmin) / (Pmax - Pmin);
u_P0 = (P1 - Pmin) / (Pmax - Pmin);
u_P1 = (P2 - Pmin) / (Pmax - Pmin);
u_P2 = (P3 - Pmin) / (Pmax - Pmin);
u_P3 = (P4 - Pmin) / (Pmax - Pmin);


% Determine the effective battery voltage from each ESC
Vb_eff_0 = u_P0 * Vb;
Vb_eff_1 = u_P1 * Vb;
Vb_eff_2 = u_P2 * Vb;
Vb_eff_3 = u_P3 * Vb;
    
Vb_eff = [Vb_eff_0, Vb_eff_1, Vb_eff_2, Vb_eff_3];
